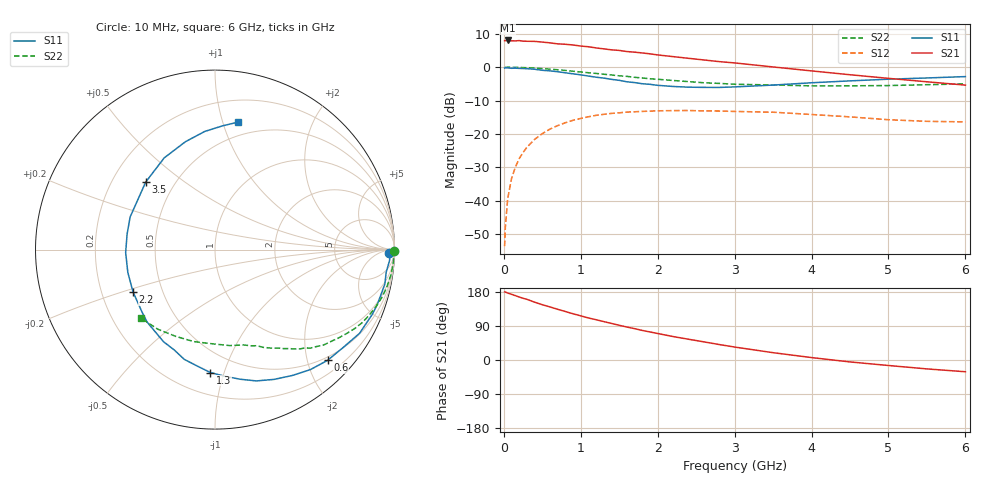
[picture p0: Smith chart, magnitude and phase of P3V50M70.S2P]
! SIEMENS Small Signal Semiconductors
! BFP181
! Si NPN RF Bipolar Junction Transistor in SOT143
! VCE = 0.5 V  IC = 0.7 mA
! Common Emitter S-Parameters:  March  1996
# GHz  S  MA  R  50
!  f  S11  S21  S12  S22
! GHz  MAG  ANG  MAG  ANG  MAG  ANG  MAG  ANG
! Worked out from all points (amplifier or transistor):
!   36 points, 10 MHz to 6 GHz, reference 50 ohm
!   highest |S21| = 8.0 dB at 50 MHz (marker M1)
!   |S21| within 3 dB of that: start of sweep to 1.506 GHz
!   unconditionally stable (mu >= 1): 2.97 GHz to end of sweep
!   at 250 MHz: K = 0.10, MSG = 16.7 dB, |S12| = -25.5 dB
!   at 1.4 GHz: K = 0.52, MSG = 9.5 dB, |S12| = -13.8 dB
!   at 6 GHz: K = 1.64, MAG = 0.8 dB, |S12| = -16.4 dB
!   S11 on the Smith chart (normalised r, x): 10 MHz: 49, -27; 600 MHz: 0.44, -2.38; 1.3 GHz: 0.35, -0.90; 2.2 GHz: 0.34, -0.22; 3.5 GHz: 0.34, +0.37; 6 GHz: 0.38, +1.12
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0.01  0.969 -1.0  2.497 179.6  0.0021 89.1  0.9986 -0.3
0.02  0.9764 -1.5  2.49 179.4  0.0041 88.1  0.9932 -0.7
0.05  0.9744 -3.6  2.508 176.7  0.0108 88.4  0.9967 -2.0
0.1  0.9619 -7.6  2.479 173.3  0.0215 83.6  0.996 -4.0
0.2  0.9581 -15.2  2.496 166.2  0.0429 79.7  0.9908 -8.0
0.4  0.9306 -30.1  2.43 152.6  0.0831 69.0  0.9684 -15.8
0.5  0.8977 -37.6  2.371 145.9  0.1014 63.8  0.9507 -19.6
0.6  0.8802 -44.4  2.31 140.0  0.1186 58.9  0.9337 -23.1
0.8  0.8228 -58.5  2.199 127.9  0.1476 50.0  0.8931 -29.6
0.9  0.7946 -65.5  2.146 122.0  0.1606 45.6  0.8691 -32.6
1.1  0.7358 -79.0  2.019 110.9  0.1811 37.6  0.8248 -38.3
1.3  0.6856 -92.1  1.877 101.3  0.197 30.2  0.7836 -43.5
1.5  0.6349 -105.7  1.78 91.6  0.2074 24.1  0.7419 -47.6
1.8  0.5651 -126.5  1.63 78.0  0.2178 16.2  0.6885 -53.2
2.2  0.5139 -152.8  1.437 61.9  0.2239 6.5  0.6318 -60.3
2.8  0.4972 170.1  1.21 40.8  0.2208 -4.7  0.5715 -69.7
3  0.5066 159.0  1.157 34.2  0.2175 -8.5  0.5553 -73.1
3.5  0.5392 135.7  1.007 19.3  0.2119 -14.5  0.5409 -81.3
4  0.5841 119.0  0.879 6.4  0.1959 -20.0  0.5251 -91.6
4.5  0.6234 105.3  0.77 -5.1  0.1804 -24.3  0.5259 -102.9
5.5  0.6891 86.9  0.604 -23.5  0.1547 -23.7  0.5462 -125.7
6  0.7223 79.7  0.539 -31.0  0.1518 -21.3  0.5623 -137.3
